FUNCTION_BLOCK Example37_ApplicationDesigner	//5x5 flyways - up to 10 xbots with the example application design loaded on the PMC as design 1
VAR_INPUT
	Execute : BOOL;
END_VAR
VAR_OUTPUT
END_VAR
VAR_IN_OUT
	PMC : PMControllerType;
END_VAR
VAR
	//System setup
	Reboot : PMC_Reboot;
	ActivatePMC : PMC_ActivateXbots;
	
	//move xbots to start
	ReadXbotIDs : PMC_ReadXbotIDs;
	i : INT;
	Home : PMC_AutoDrivingMotion;
	XbotIndex : USINT;
	SendToStart : PMC_App_SendXbotToStation;
	
	//station 1 bay 1
	HoldForXbot_Station1Bay1 : PMC_App_HoldForBay;
	SelectNextBay_Station1Bay1 : PseudoRandom;
	SendToNextBay_Station1Bay1 : PMC_App_SendXbotToStation;
	
	//station 1 bay 2
	HoldForXbot_Station1Bay2 : PMC_App_HoldForBay;
	SelectNextBay_Station1Bay2 : PseudoRandom;
	SendToNextBay_Station1Bay2 : PMC_App_SendXbotToStation;
	
	//station 2 bay 1
	HoldForXbot_Station2Bay1 : PMC_App_HoldForBay;
	SelectNextBay_Station2Bay1 : PseudoRandom;
	SendToNextBay_Station2Bay1 : PMC_App_SendXbotToStation;
	
	//station 2 bay 2
	HoldForXbot_Station2Bay2 : PMC_App_HoldForBay;
	SelectNextBay_Station2Bay2 : PseudoRandom;
	SendToNextBay_Station2Bay2 : PMC_App_SendXbotToStation;
END_VAR

//5x5 flyways, up to 10 xbots - example application design loaded on the PMC as design 1

IF NOT Execute THEN
	XbotIndex := 0;
END_IF;

//start the system
Reboot(Execute := Execute,PM_Controller := PMC);
ActivatePMC(Execute := Reboot.Done,PM_Controller := PMC);

//move xbots to starting positions
ReadXbotIDs(Enable := ActivatePMC.Done,PM_Controller := PMC);
FOR i := 0 TO 9 DO
	Home.XbotID[i] := INT_TO_USINT(i + 1);
	Home.PosX[i] := 0.06 + 0.12*i;
	Home.PosY[i] := 0.06;
END_FOR;
Home(Execute := ReadXbotIDs.Valid,nXbots := ReadXbotIDs.NumXbots,PM_Controller := PMC);
SendToStart(Execute := Home.Done,XbotID := XbotIndex + 1,StationID := 1,BayID := 1,PM_Controller := PMC);
IF SendToStart.Ack AND XbotIndex + 1 < ReadXbotIDs.NumXbots THEN
	XbotIndex := XbotIndex + 1;
	SendToStart(Execute := FALSE,PM_Controller := PMC);
END_IF;

//station 1 bay 1
HoldForXbot_Station1Bay1(Execute := SendToStart.Ack,StationID := 1,BayID := 1,PM_Controller := PMC);
SelectNextBay_Station1Bay1(Execute := HoldForXbot_Station1Bay1.Done,Seed := 11);
SendToNextBay_Station1Bay1(Execute := HoldForXbot_Station1Bay1.Done,XbotID := HoldForXbot_Station1Bay1.XbotID,StationID := 2,BayID := UDINT_TO_USINT(SelectNextBay_Station1Bay1.RandomNumber MOD 2) + 1,PM_Controller := PMC);
IF SendToNextBay_Station1Bay1.Ack THEN
	HoldForXbot_Station1Bay1(Execute := FALSE,PM_Controller := PMC);
	SelectNextBay_Station1Bay1(Execute := FALSE);
	SendToNextBay_Station1Bay1(Execute := FALSE,PM_Controller := PMC);
END_IF;

//station 1 bay 2
HoldForXbot_Station1Bay2(Execute := SendToStart.Ack,StationID := 1,BayID := 2,PM_Controller := PMC);
SelectNextBay_Station1Bay2(Execute := HoldForXbot_Station1Bay2.Done,Seed := 12);
SendToNextBay_Station1Bay2(Execute := HoldForXbot_Station1Bay2.Done,XbotID := HoldForXbot_Station1Bay2.XbotID,StationID := 2,BayID := UDINT_TO_USINT(SelectNextBay_Station1Bay2.RandomNumber MOD 2) + 1,PM_Controller := PMC);
IF SendToNextBay_Station1Bay2.Ack THEN
	HoldForXbot_Station1Bay2(Execute := FALSE,PM_Controller := PMC);
	SelectNextBay_Station1Bay2(Execute := FALSE);
	SendToNextBay_Station1Bay2(Execute := FALSE,PM_Controller := PMC);
END_IF;

//station 2 bay 1
HoldForXbot_Station2Bay1(Execute := SendToStart.Ack,StationID := 2,BayID := 1,PM_Controller := PMC);
SelectNextBay_Station2Bay1(Execute := HoldForXbot_Station2Bay1.Done,Seed := 21);
SendToNextBay_Station2Bay1(Execute := HoldForXbot_Station2Bay1.Done,XbotID := HoldForXbot_Station2Bay1.XbotID,StationID := 1,BayID := UDINT_TO_USINT(SelectNextBay_Station2Bay1.RandomNumber MOD 2) + 1,PM_Controller := PMC);
IF SendToNextBay_Station2Bay1.Ack THEN
	HoldForXbot_Station2Bay1(Execute := FALSE,PM_Controller := PMC);
	SelectNextBay_Station2Bay1(Execute := FALSE);
	SendToNextBay_Station2Bay1(Execute := FALSE,PM_Controller := PMC);
END_IF;

//station 2 bay 2
HoldForXbot_Station2Bay2(Execute := SendToStart.Ack,StationID := 2,BayID := 2,PM_Controller := PMC);
SelectNextBay_Station2Bay2(Execute := HoldForXbot_Station2Bay2.Done,Seed := 22);
SendToNextBay_Station2Bay2(Execute := HoldForXbot_Station2Bay2.Done,XbotID := HoldForXbot_Station2Bay2.XbotID,StationID := 1,BayID := UDINT_TO_USINT(SelectNextBay_Station2Bay2.RandomNumber MOD 2) + 1,PM_Controller := PMC);
IF SendToNextBay_Station2Bay2.Ack THEN
	HoldForXbot_Station2Bay2(Execute := FALSE,PM_Controller := PMC);
	SelectNextBay_Station2Bay2(Execute := FALSE);
	SendToNextBay_Station2Bay2(Execute := FALSE,PM_Controller := PMC);
END_IF;

END_FUNCTION_BLOCK
